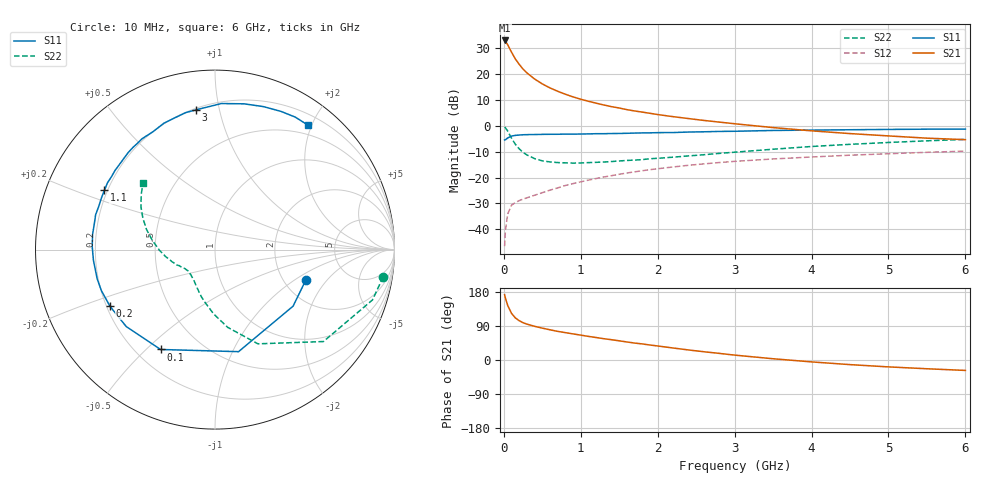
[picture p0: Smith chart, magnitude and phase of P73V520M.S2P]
! SIEMENS Small Signal Semiconductors
! BFP196
! Si NPN RF Bipolar Junction Transistor in SOT143
! VCE = 3.5 V  IC = 20 mA
! Common Emitter S-Parameters:  May  1996
# GHz  S  MA  R  50
!  f  S11  S21  S12  S22
! GHz  MAG  ANG  MAG  ANG  MAG  ANG  MAG  ANG
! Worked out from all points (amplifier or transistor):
!   36 points, 10 MHz to 6 GHz, reference 50 ohm
!   highest |S21| = 33.1 dB at 10 MHz (marker M1)
!   |S21| within 3 dB of that: start of sweep to 73.31 MHz
!   unconditionally stable (mu >= 1): 672.1 MHz to 3.427 GHz
!   at 250 MHz: K = 0.60, MSG = 25.2 dB, |S12| = -28.3 dB
!   at 1.4 GHz: K = 1.11, MAG = 11.3 dB, |S12| = -19.3 dB
!   at 6 GHz: K = 0.96, MSG = 2.2 dB, |S12| = -9.8 dB
!   S11 on the Smith chart (normalised r, x): 10 MHz: 2.61, -1.25; 100 MHz: 0.30, -0.55; 200 MHz: 0.21, -0.24; 1.1 GHz: 0.19, +0.24; 3 GHz: 0.21, +0.85; 6 GHz: 0.35, +1.94
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0.01  0.5337 -18.7  44.94 172.3  0.0047 84.1  0.9491 -9.2
0.02  0.5371 -35.9  43.26 163.6  0.0093 77.0  0.9214 -17.7
0.05  0.5836 -77.0  37.14 144.0  0.0197 61.0  0.7921 -40.3
0.1  0.6338 -118.6  26.64 123.0  0.0292 46.7  0.5769 -65.5
0.15  0.6545 -139.1  19.68 111.0  0.0329 41.3  0.4391 -80.7
0.2  0.6648 -151.6  15.48 103.7  0.0358 40.7  0.3593 -91.1
0.25  0.673 -160.1  12.55 98.4  0.0383 40.7  0.3054 -99.5
0.3  0.6763 -166.1  10.6 94.6  0.0405 42.2  0.2741 -106.0
0.4  0.6799 -174.9  8.065 88.9  0.0455 45.2  0.2325 -116.0
0.5  0.6843 178.6  6.48 84.1  0.0509 47.2  0.2105 -123.3
0.6  0.6872 173.0  5.42 79.7  0.0571 49.3  0.2006 -128.9
0.7  0.6878 167.7  4.669 75.6  0.063 51.1  0.1949 -133.5
0.9  0.691 159.7  3.633 68.9  0.0763 52.6  0.1903 -140.0
1.1  0.699 151.8  2.989 62.3  0.0892 52.8  0.1946 -144.4
1.3  0.7054 144.7  2.534 56.2  0.1025 52.0  0.1996 -148.6
1.6  0.7181 135.0  2.059 47.6  0.1223 50.2  0.2142 -153.9
2.2  0.7422 117.7  1.507 31.7  0.1602 44.1  0.2478 -163.9
3  0.7859 97.7  1.099 12.9  0.2056 34.4  0.3094 -179.3
3.5  0.8145 87.5  0.926 3.3  0.2289 28.2  0.3531 171.6
4.5  0.8413 71.2  0.709 -12.2  0.2707 16.8  0.4392 156.3
5.5  0.863 58.8  0.578 -23.1  0.3074 6.0  0.5135 143.2
6  0.8654 53.4  0.541 -27.5  0.3246 0.1  0.5468 137.0
